PROGRAM AlarmsAndEvents
VAR
	isInitialized      : BOOL := FALSE;
	sendInfo           : BOOL := FALSE;
	sendWarning        : BOOL := FALSE;
	raiseAlarmError    : BOOL := FALSE;
	raiseAlarmWarning  : BOOL := FALSE;
	confirmAlarmError  : BOOL;
	clearAlarms        : BOOL;
	fbMessageInfo      : FB_TcMessage;
	fbMessageWarning   : FB_TcMessage;	
	fbAlarmWarning     : FB_TcAlarm;		
	fbAlarmError       : FB_TcAlarm;	
END_VAR

// This code demonstrates usage of EventLogger system for Alarms and Events.
// However, CX7000 PLC is not capable of using EventLogger. Thus we need workarounds. See PRG AlarmsAndEventsCX7000.

IF NOT isInitialized THEN
	isInitialized := TRUE;
	fbMessageInfo.CreateEx(TC_EVENTS.MyEventClass.MyEventInfo, 0);
	fbMessageWarning.CreateEx(TC_EVENTS.MyEventClass.MyEventWarning, 0);
	fbAlarmWarning.CreateEx(TC_EVENTS.MyEventClass.MyEventWarning, 0, 0);
	fbAlarmError.CreateEx(TC_EVENTS.MyEventClass.MyEventError, 1, 0);
END_IF

IF sendInfo THEN
	sendInfo := FALSE;
	fbMessageInfo.Send(0); // 0 - set current timestamp automatically
END_IF

IF sendWarning THEN
	sendWarning := FALSE;
	fbMessageWarning.Send(0);
END_IF

IF raiseAlarmWarning THEN
	raiseAlarmWarning := FALSE;
	fbAlarmWarning.Raise(0);
END_IF

IF raiseAlarmError THEN
	raiseAlarmError := FALSE;
	fbAlarmError.Raise(0);
END_IF

IF confirmAlarmError THEN
	confirmAlarmError := FALSE;
	fbAlarmError.Confirm(0);
END_IF

IF clearAlarms THEN
	clearAlarms := FALSE;
	fbAlarmWarning.Clear(0, TRUE);
	fbAlarmError.Clear(0, TRUE);
END_IF

END_PROGRAM
